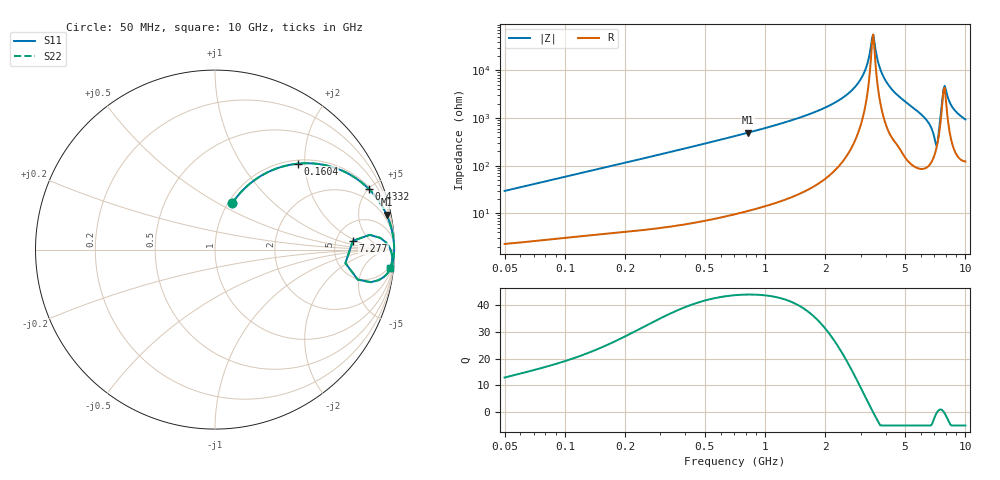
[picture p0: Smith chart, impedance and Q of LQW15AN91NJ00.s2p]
!Murata Part Number: LQW15AN91NJ00
!These Parameters are Measured in Series Mode Connection
!  o--[Z]--o
!Port1  Port2
!  o-------o
!Freq. Start=50[MHz] Stop=10[GHz], 401[Steps]
# Hz S RI R 50
!Freq.(Hz)	S 11(Real)	S 11(Imag)	S 21(Real)	S 21(Imag)	S 12(Real)	S 12(Imag)	S 22(Real)	S 22(Imag)
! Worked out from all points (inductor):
!   401 points, 50 MHz to 10 GHz, reference 50 ohm
!   read as one part in series: L = 93 nH near 51.34 MHz
!   highest Q = 43.9 at 818 MHz (marker M1), where L = 94.9 nH
!   self-resonance near 3.42 GHz
!   S11 on the Smith chart (normalised r, x): 50 MHz: 1.05, +0.59; 160.4 MHz: 1.07, +1.85; 433.2 MHz: 1.12, +5.00; 7.277 GHz: 7.26, +1.75; 10 GHz: 3, -18
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5e7  0.0966 0.2592  0.9034 -0.2592  0.9034 -0.2592  0.0966 0.2592
1.214486e8  0.3375 0.4499  0.6625 -0.4499  0.6625 -0.4499  0.3375 0.4499
1.603971e8  0.4618 0.4788  0.5382 -0.4788  0.5382 -0.4788  0.4618 0.4788
2.949953e8  0.7355 0.4269  0.2645 -0.4269  0.2645 -0.4269  0.7355 0.4269
4.331514e8  0.8558 0.3391  0.1442 -0.3391  0.1442 -0.3391  0.8558 0.3391
7.071068e8  0.9409 0.2246  0.0591 -0.2246  0.0591 -0.2246  0.9409 0.2246
8.180189e8  0.9556 0.1948  0.0444 -0.1948  0.0444 -0.1948  0.9556 0.1948
1.717543e9  0.9916 0.0783  0.00835 -0.0783  0.00835 -0.0783  0.9916 0.0783
2.298604e9  0.9963 0.0441  0.00373 -0.0441  0.00373 -0.0441  0.9963 0.0441
2.803837e9  0.9978 0.0225  0.00218 -0.0225  0.00218 -0.0225  0.9978 0.0225
3.117263e9  0.9982 0.0112  0.00181 -0.0112  0.00181 -0.0112  0.9982 0.0112
3.465724e9  0.9982 -0.000275  0.00175 0.000275  0.00175 0.000275  0.9982 -0.000275
3.802437e9  0.998 -0.0106  0.00201 0.0106  0.00201 0.0106  0.998 -0.0106
4.171863e9  0.9973 -0.0215  0.0027 0.0215  0.0027 0.0215  0.9973 -0.0215
6.207365e9  0.9833 -0.0931  0.0167 0.0931  0.0167 0.0931  0.9833 -0.0931
6.901252e9  0.9126 -0.1698  0.0874 0.1698  0.0874 0.1698  0.9126 -0.1698
7.086521e9  0.7954 -0.1672  0.2046 0.1672  0.2046 0.1672  0.7954 -0.1672
7.276762e9  0.7684 0.0491  0.2316 -0.0491  0.2316 -0.0491  0.7684 0.0491
7.672705e9  0.9674 0.0208  0.0326 -0.0208  0.0326 -0.0208  0.9674 0.0208
7.878683e9  0.9809 -0.00837  0.0191 0.00837  0.0191 0.00837  0.9809 -0.00837
8.759398e9  0.9863 -0.0635  0.0137 0.0635  0.0137 0.0635  0.9863 -0.0635
1e10  0.9752 -0.1027  0.0248 0.1027  0.0248 0.1027  0.9752 -0.1027
